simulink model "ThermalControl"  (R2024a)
settings: Solver=FixedStepDiscrete  StartTime=0.0  StopTime=10000  FixedStep=0.1  RelTol=1e-3
undefined symbols (not defined in the file): CtrlThrBattTrgTemp, CtrlThrEMTrgTemp
libraries: simulink x1

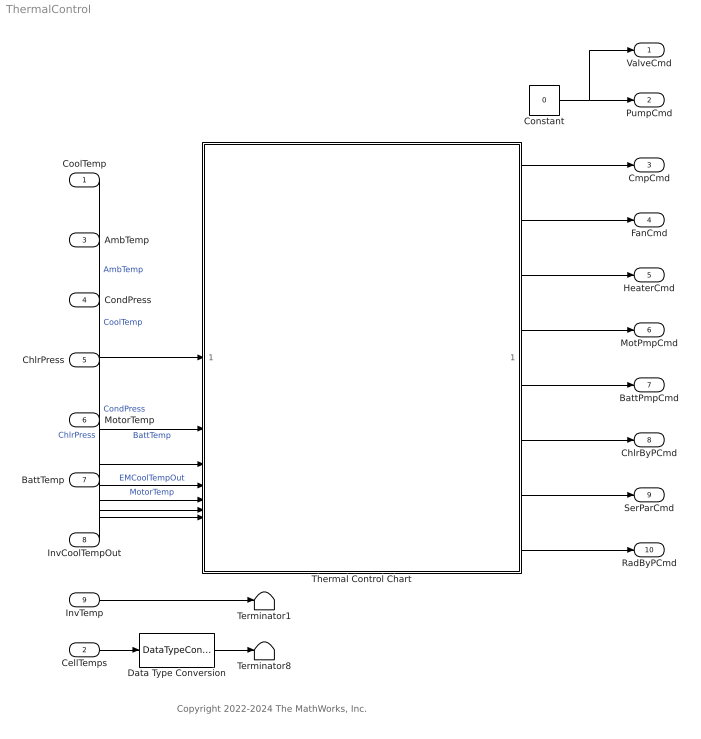
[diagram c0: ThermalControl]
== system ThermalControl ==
  note: Copyright 2022-2024 The MathWorks, Inc.
  CoolTemp : Inport  Unit=K
  CellTemps : Inport  Port=2  PortDimensions=PlntBattNumCellSer
  AmbTemp : Inport  Port=3  Unit=K
  CondPress : Inport  Port=4  Unit=MPa
  ChlrPress : Inport  Port=5  Unit=MPa
  MotorTemp : Inport  Port=6  Unit=K
  BattTemp : Inport  Port=7  Unit=K
  InvCoolTempOut : Inport  Port=8  Unit=K
  InvTemp : Inport  Port=9  Unit=K
  Constant : Constant  Value=0  SampleTime=0.1
  Data Type Conversion : DataTypeConversion  OutDataTypeStr=single
  Terminator1 : Terminator
  Terminator8 : Terminator
  Thermal Control Chart : Stateflow chart  TreatAsAtomicUnit=on
  ValveCmd : Outport
  PumpCmd : Outport  Port=2
  CmpCmd : Outport  Port=3
  FanCmd : Outport  Port=4
  HeaterCmd : Outport  Port=5
  MotPmpCmd : Outport  Port=6
  BattPmpCmd : Outport  Port=7
  ChlrByPCmd : Outport  Port=8
  SerParCmd : Outport  Port=9
  RadByPCmd : Outport  Port=10
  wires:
  AmbTemp/1 -> Thermal Control Chart/1(AmbTemp)  "AmbTemp"
  CondPress/1 -> Thermal Control Chart/7(CondPress)  "CondPress"
  BattTemp/1 -> Thermal Control Chart/2(BattTemp)  "BattTemp"
  InvCoolTempOut/1 -> Thermal Control Chart/4(EMCoolTempOut)  "EMCoolTempOut"
  CoolTemp/1 -> Thermal Control Chart/3(CoolTemp)  "CoolTemp"
  MotorTemp/1 -> Thermal Control Chart/5(MotorTemp)  "MotorTemp"
  Thermal Control Chart/1(BattPmpCmd) -> BattPmpCmd/1
  Thermal Control Chart/2(ChlrByPCmd) -> ChlrByPCmd/1
  Thermal Control Chart/5(MotPmpCmd) -> MotPmpCmd/1
  Thermal Control Chart/4(SerParCmd) -> SerParCmd/1
  Thermal Control Chart/3(RadByPCmd) -> RadByPCmd/1
  Thermal Control Chart/6(HeaterCmd) -> HeaterCmd/1
  Thermal Control Chart/7(CmpCmd) -> CmpCmd/1
  ChlrPress/1 -> Thermal Control Chart/6(ChlrPress)  "ChlrPress"
  Thermal Control Chart/8(FanCmd) -> FanCmd/1
  Constant/1 -> ValveCmd/1, PumpCmd/1
  Data Type Conversion/1 -> Terminator8/1
  CellTemps/1 -> Data Type Conversion/1
  InvTemp/1 -> Terminator1/1

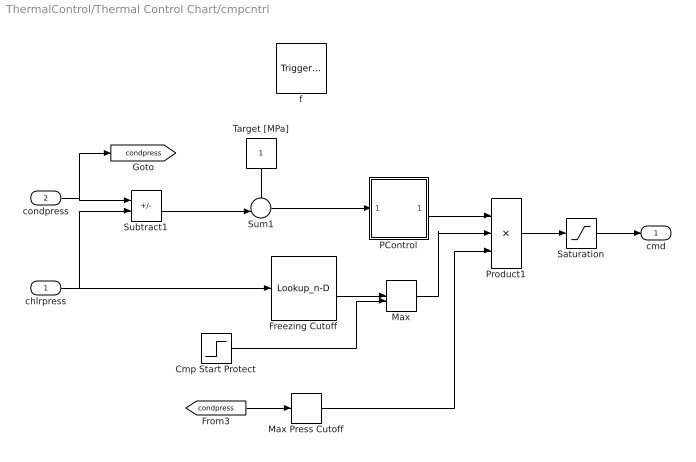
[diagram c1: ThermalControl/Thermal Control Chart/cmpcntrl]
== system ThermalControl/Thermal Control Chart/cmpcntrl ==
  chlrpress : Inport  OutDataTypeStr=double  PortDimensions=1
  condpress : Inport  Port=2  OutDataTypeStr=double  PortDimensions=1
  f : TriggerPort  TriggerType=function-call  VariantControl=(inherit)  SampleTime=-1
  Cmp Start Protect : Step  Time=15  Before=1  After=0
  Freezing Cutoff : Lookup_n-D  NumberOfTableDimensions=1  BreakpointsForDimension1=[0.3 0.31]  IndexSearchMethod=Linear search  BeginIndexSearchUsingPreviousIndexResult=on  Table=[0.1 1]  ExtrapMethod=Clip  InternalRulePriority=Speed  RndMeth=Simplest
  Max : MinMax  Function=max  Inputs=2
  Max Press Cutoff : Relay  OnSwitchValue=3  OffSwitchValue=2.9  OnOutputValue=0.1  OffOutputValue=1
  PControl : Subsystem
  Product1 : Product  Inputs=3
  Saturation : Saturate  UpperLimit=1  LowerLimit=0.1
  Subtract1 : Sum  Inputs=+-
  Sum1 : Sum  Inputs=+-|
  Target [MPa] : Constant
  cmd : Outport
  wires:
  Target [MPa]/1 -> Sum1/1
  Cmp Start Protect/1 -> Max/2
  Max/1 -> Product1/2
  Saturation/1 -> cmd/1
  PControl/1(cmd) -> Product1/1
  [condpress] -> Max Press Cutoff/1
  Max Press Cutoff/1 -> Product1/3
  Freezing Cutoff/1 -> Max/1
  Sum1/1 -> PControl/1(input)
  Product1/1 -> Saturation/1
  Subtract1/1 -> Sum1/2
  condpress/1 -> [condpress], Subtract1/1
  chlrpress/1 -> Subtract1/2, Freezing Cutoff/1

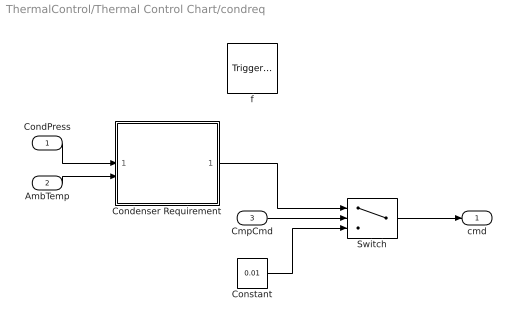
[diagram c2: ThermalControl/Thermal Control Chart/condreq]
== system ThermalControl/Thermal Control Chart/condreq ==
  CondPress : Inport  OutDataTypeStr=double  PortDimensions=1
  AmbTemp : Inport  Port=2  OutDataTypeStr=double  PortDimensions=1
  CmpCmd : Inport  Port=3  OutDataTypeStr=double  PortDimensions=1
  f : TriggerPort  TriggerType=function-call  VariantControl=(inherit)  SampleTime=-1
  Condenser Requirement : Subsystem
  Constant : Constant  Value=0.01  SampleTime=-1
  Switch : Switch  Criteria=u2 > Threshold
  cmd : Outport
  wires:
  Switch/1 -> cmd/1
  Constant/1 -> Switch/3
  CmpCmd/1 -> Switch/2
  Condenser Requirement/1(cmd_fan) -> Switch/1
  CondPress/1 -> Condenser Requirement/1(p_cond)
  AmbTemp/1 -> Condenser Requirement/2(T_env)

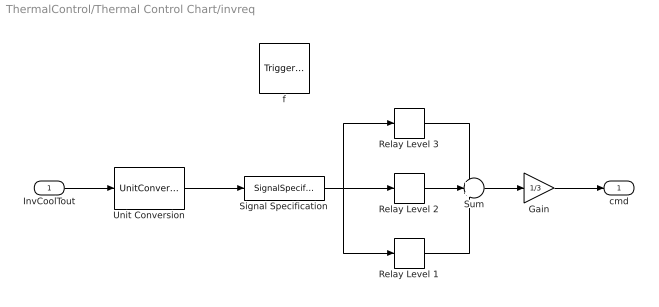
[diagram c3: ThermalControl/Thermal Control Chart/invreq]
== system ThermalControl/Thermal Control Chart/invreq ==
  InvCoolTout : Inport  OutDataTypeStr=double  Unit=K  PortDimensions=1
  f : TriggerPort  TriggerType=function-call  VariantControl=(inherit)  SampleTime=-1
  Gain : Gain  Gain=1/3
  Relay Level 1 : Relay  OnSwitchValue=75  OffSwitchValue=65
  Relay Level 2 : Relay  OnSwitchValue=85  OffSwitchValue=76
  Relay Level 3 : Relay  OnSwitchValue=95  OffSwitchValue=86
  Signal Specification : SignalSpecification  Unit=°C
  Sum : Sum  Inputs=+++
  Unit Conversion : UnitConversion
  cmd : Outport
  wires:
  Relay Level 2/1 -> Sum/2
  Sum/1 -> Gain/1
  Signal Specification/1 -> Relay Level 2/1, Relay Level 3/1, Relay Level 1/1
  Relay Level 1/1 -> Sum/3
  Relay Level 3/1 -> Sum/1
  Unit Conversion/1 -> Signal Specification/1
  Gain/1 -> cmd/1
  InvCoolTout/1 -> Unit Conversion/1

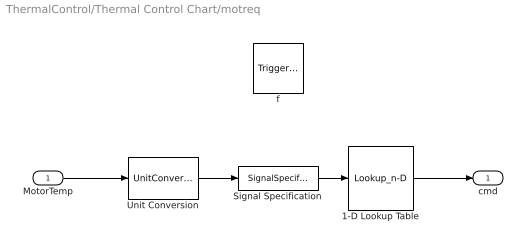
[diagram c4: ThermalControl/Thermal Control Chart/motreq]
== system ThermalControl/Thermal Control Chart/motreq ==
  MotorTemp : Inport  OutDataTypeStr=double  Unit=K  PortDimensions=1
  f : TriggerPort  TriggerType=function-call  VariantControl=(inherit)  SampleTime=-1
  1-D Lookup Table : Lookup_n-D  NumberOfTableDimensions=1  BreakpointsForDimension1=[-50 45 48 52 58 60 75 130]  IndexSearchMethod=Linear search  BeginIndexSearchUsingPreviousIndexResult=on  Table=[0 0 0.1 0.3 0.5 0.7 1 1]  InternalRulePriority=Speed  RndMeth=Simplest
  Signal Specification : SignalSpecification  Unit=°C
  Unit Conversion : UnitConversion
  cmd : Outport
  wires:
  Unit Conversion/1 -> Signal Specification/1
  Signal Specification/1 -> 1-D Lookup Table/1
  1-D Lookup Table/1 -> cmd/1
  MotorTemp/1 -> Unit Conversion/1

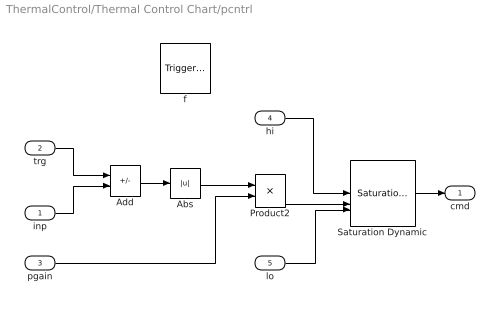
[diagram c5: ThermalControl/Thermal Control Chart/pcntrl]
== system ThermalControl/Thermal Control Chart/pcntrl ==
  inp : Inport  OutDataTypeStr=double  PortDimensions=1
  trg : Inport  Port=2  OutDataTypeStr=double  PortDimensions=1
  pgain : Inport  Port=3  OutDataTypeStr=double  PortDimensions=1
  hi : Inport  Port=4  OutDataTypeStr=double  PortDimensions=1
  lo : Inport  Port=5  OutDataTypeStr=double  PortDimensions=1
  f : TriggerPort  TriggerType=function-call  VariantControl=(inherit)  SampleTime=-1
  Abs : Abs
  Add : Sum  Inputs=+-
  Product2 : Product
  Saturation Dynamic : simulink/Discontinuities/Saturation Dynamic  OutMin=[]  OutMax=[]  OutDataTypeStr=Inherit: Same as second input  OutDataType=fixdt(1, 16)  OutScaling=2^-10  DoSatur=off
  cmd : Outport
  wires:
  trg/1 -> Add/1
  inp/1 -> Add/2
  Add/1 -> Abs/1
  Saturation Dynamic/1 -> cmd/1
  pgain/1 -> Product2/2
  Product2/1 -> Saturation Dynamic/2
  Abs/1 -> Product2/1
  hi/1 -> Saturation Dynamic/1
  lo/1 -> Saturation Dynamic/3

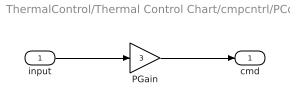
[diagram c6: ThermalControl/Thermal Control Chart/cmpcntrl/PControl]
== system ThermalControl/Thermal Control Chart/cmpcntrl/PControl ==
  input : Inport
  PGain : Gain  Gain=3
  cmd : Outport
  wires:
  input/1 -> PGain/1
  PGain/1 -> cmd/1

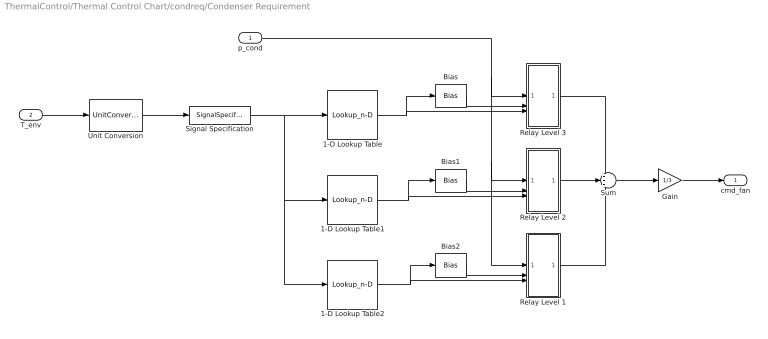
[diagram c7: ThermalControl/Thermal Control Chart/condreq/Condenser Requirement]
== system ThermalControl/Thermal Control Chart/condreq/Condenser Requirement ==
  p_cond : Inport
  T_env : Inport  Port=2  Unit=K
  1-D Lookup Table : Lookup_n-D  NumberOfTableDimensions=1  BreakpointsForDimension1=[0 20 30 40 50]  IndexSearchMethod=Linear search  BeginIndexSearchUsingPreviousIndexResult=on  Table=[2.0 2.0 1.8 1.5 1.3]  InternalRulePriority=Speed  RndMeth=Simplest
  1-D Lookup Table1 : Lookup_n-D  NumberOfTableDimensions=1  BreakpointsForDimension1=[0 20 30 40 50]  IndexSearchMethod=Linear search  BeginIndexSearchUsingPreviousIndexResult=on  Table=[1.4 1.4 1.3 1.2 1.1]  InternalRulePriority=Speed  RndMeth=Simplest
  1-D Lookup Table2 : Lookup_n-D  NumberOfTableDimensions=1  BreakpointsForDimension1=[0 20 30 40 50]  IndexSearchMethod=Linear search  BeginIndexSearchUsingPreviousIndexResult=on  Table=[0.8 0.8 0.8 0.8 0.8]  InternalRulePriority=Speed  RndMeth=Simplest
  Bias : Bias  Bias=0.4
  Bias1 : Bias  Bias=0.4
  Bias2 : Bias  Bias=0.3
  Gain : Gain  Gain=1/3
  Relay Level 1 : Subsystem
  Relay Level 2 : Subsystem
  Relay Level 3 : Subsystem
  Signal Specification : SignalSpecification  Unit=°C
  Sum : Sum  Inputs=+++
  Unit Conversion : UnitConversion
  cmd_fan : Outport
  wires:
  Unit Conversion/1 -> Signal Specification/1
  Signal Specification/1 -> 1-D Lookup Table2/1, 1-D Lookup Table1/1, 1-D Lookup Table/1
  Gain/1 -> cmd_fan/1
  T_env/1 -> Unit Conversion/1
  Bias2/1 -> Relay Level 1/2(high)
  1-D Lookup Table2/1 -> Bias2/1, Relay Level 1/3(low)
  Bias1/1 -> Relay Level 2/2(high)
  1-D Lookup Table1/1 -> Bias1/1, Relay Level 2/3(low)
  Bias/1 -> Relay Level 3/2(high)
  1-D Lookup Table/1 -> Bias/1, Relay Level 3/3(low)
  Relay Level 1/1(out) -> Sum/3
  Relay Level 2/1(out) -> Sum/2
  Relay Level 3/1(out) -> Sum/1
  p_cond/1 -> Relay Level 1/1(in), Relay Level 2/1(in), Relay Level 3/1(in)
  Sum/1 -> Gain/1

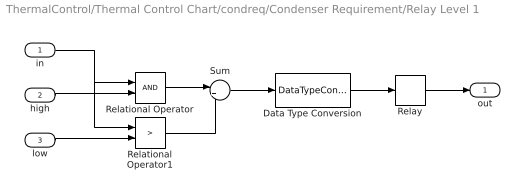
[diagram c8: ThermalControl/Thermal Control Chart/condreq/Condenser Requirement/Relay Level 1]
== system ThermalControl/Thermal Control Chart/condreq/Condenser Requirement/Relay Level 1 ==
  in : Inport
  high : Inport  Port=2
  low : Inport  Port=3
  Data Type Conversion : DataTypeConversion
  Relational Operator : RelationalOperator  OutDataTypeStr=boolean  RndMeth=Simplest
  Relational Operator1 : RelationalOperator  Operator=>  OutDataTypeStr=boolean  RndMeth=Simplest
  Relay : Relay  OnSwitchValue=1.5  OffSwitchValue=0.5
  Sum : Sum  Inputs=|++
  out : Outport
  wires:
  in/1 -> Relational Operator1/1, Relational Operator/1
  high/1 -> Relational Operator/2
  low/1 -> Relational Operator1/2
  Relay/1 -> out/1
  Relational Operator/1 -> Sum/1
  Relational Operator1/1 -> Sum/2
  Data Type Conversion/1 -> Relay/1
  Sum/1 -> Data Type Conversion/1

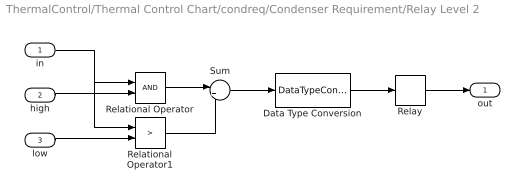
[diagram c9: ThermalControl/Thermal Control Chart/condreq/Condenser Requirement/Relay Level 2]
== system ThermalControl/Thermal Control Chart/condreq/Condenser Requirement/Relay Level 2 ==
  in : Inport
  high : Inport  Port=2
  low : Inport  Port=3
  Data Type Conversion : DataTypeConversion
  Relational Operator : RelationalOperator  OutDataTypeStr=boolean  RndMeth=Simplest
  Relational Operator1 : RelationalOperator  Operator=>  OutDataTypeStr=boolean  RndMeth=Simplest
  Relay : Relay  OnSwitchValue=1.5  OffSwitchValue=0.5
  Sum : Sum  Inputs=|++
  out : Outport
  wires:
  in/1 -> Relational Operator1/1, Relational Operator/1
  high/1 -> Relational Operator/2
  low/1 -> Relational Operator1/2
  Relay/1 -> out/1
  Relational Operator/1 -> Sum/1
  Relational Operator1/1 -> Sum/2
  Data Type Conversion/1 -> Relay/1
  Sum/1 -> Data Type Conversion/1

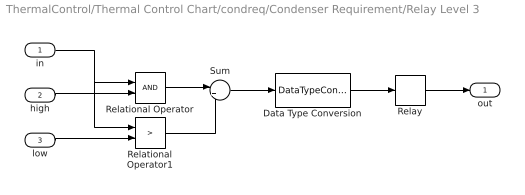
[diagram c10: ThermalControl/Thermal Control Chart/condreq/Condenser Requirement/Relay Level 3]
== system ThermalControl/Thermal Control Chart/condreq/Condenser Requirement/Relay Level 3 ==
  in : Inport
  high : Inport  Port=2
  low : Inport  Port=3
  Data Type Conversion : DataTypeConversion
  Relational Operator : RelationalOperator  OutDataTypeStr=boolean  RndMeth=Simplest
  Relational Operator1 : RelationalOperator  Operator=>  OutDataTypeStr=boolean  RndMeth=Simplest
  Relay : Relay  OnSwitchValue=1.5  OffSwitchValue=0.5
  Sum : Sum  Inputs=|++
  out : Outport
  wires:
  in/1 -> Relational Operator1/1, Relational Operator/1
  high/1 -> Relational Operator/2
  low/1 -> Relational Operator1/2
  Relay/1 -> out/1
  Relational Operator/1 -> Sum/1
  Relational Operator1/1 -> Sum/2
  Data Type Conversion/1 -> Relay/1
  Sum/1 -> Data Type Conversion/1

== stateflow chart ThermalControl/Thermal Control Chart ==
  state Pumps [parallel]
    state PumpsON
      during:
      BattPmpCmd = ...
      pcntrl(BattTemp,CtrlThrBattTrgTemp,1,1,0.1);
    state PumpsOFF
      entry:
      BattPmpCmd = 0.01;
    (default) -> PumpsOFF
    PumpsOFF -> PumpsON : [BattTemp - CtrlThrBattTrgTemp > 0 || MotorTemp - CtrlThrEMTrgTemp > 3 || ...  CtrlThrBattTrgTemp - AmbTemp > 20]
    PumpsON -> PumpsOFF : [CtrlThrBattTrgTemp - BattTemp > 5 && CtrlThrEMTrgTemp - MotorTemp > 5]
  state Heater [parallel]
    state HeatON
      entry:
      HeaterCmd = 1;
    state HeatOFF
      entry:
      HeaterCmd = 0;
    (default) -> HeatOFF
    HeatOFF -> HeatON : [BattPmpCmd > 0 && CtrlThrBattTrgTemp - CoolTemp > 20 && ... CtrlThrBattTrgTemp - AmbTemp > 20 ]
    HeatON -> HeatOFF : [CtrlThrBattTrgTemp - CoolTemp < 10]
  state cmd = pcntrl(inp,trg,pgain,hi,lo) [function]
  state cmd = cmpcntrl(chlrpress, ... [function]
    condpress)
  state ChillerBypass [parallel]
    state ChillerON
      entry:
      ChlrByPCmd = 0;
      during:
      CmpCmd = ...
      cmpcntrl(ChlrPress,CondPress);
    state ChillerOFF
      entry:
      ChlrByPCmd = 1;
      CmpCmd = 0;
    (default) -> ChillerOFF
    ChillerOFF -> ChillerON : [HeaterCmd == 0 && BattPmpCmd > 0.01 && ...  BattTemp - CtrlThrBattTrgTemp > 0 && ... BattTemp - CoolTemp < 5]
    ChillerON -> ChillerOFF : [CtrlThrBattTrgTemp - BattTemp > 5 ]
  state cmd = condreq(CondPress, ... [function]
    AmbTemp,CmpCmd)
  state cmd = invreq(InvCoolTout) [function]
  state RadiatorBypass [parallel]
    state RadiatorON
      entry:
      RadByPCmd = 0;
      during:
      fcmd1 = condreq(CondPress,AmbTemp,CmpCmd);
      fcmd2 = invreq(EMCoolTempOut);
      fcmd3 = motreq(MotorTemp);
      FanCmd = max([fcmd1,fcmd2,fcmd3]);
    state RadiatorOFF
      entry:
      RadByPCmd = 1;
      during:
      FanCmd = condreq(CondPress,AmbTemp,CmpCmd);
    (default) -> RadiatorOFF
    RadiatorOFF -> RadiatorON : [HeaterCmd == 0 && BattPmpCmd > 0 && ... EMCoolTempOut - CtrlThrEMTrgTemp > 0 && ... EMCoolTempOut - AmbTemp > 0]
    RadiatorON -> RadiatorOFF : [AmbTemp - EMCoolTempOut > 0]
  state cmd = motreq(MotorTemp) [function]
  state SeriesParallel [parallel]
    state Parallel
      entry:
      SerParCmd = 0;
      during:
      MotPmpCmd = ...
      pcntrl(MotorTemp,CtrlThrEMTrgTemp,1,1,0.1);
    state Series
      entry:
      SerParCmd = 1;
      during:
      MotPmpCmd = BattPmpCmd;
    (default) -> Series
    Series -> Parallel : [BattPmpCmd > 0.01 && (ChlrByPCmd < 0.5 || ... max(AmbTemp,EMCoolTempOut) - CtrlThrBattTrgTemp > 10 ... || MotorTemp - BattTemp > 50)]
    Parallel -> Series : [max(AmbTemp,EMCoolTempOut) - CtrlThrBattTrgTemp < 5]
  data: inp function_input double; trg function_input double; pgain function_input double; hi function_input double; lo function_input double; cmd function_output; chlrpress function_input double; condpress function_input double; cmd function_output; CondPress function_input double; AmbTemp function_input double; CmpCmd function_input double; cmd function_output; InvCoolTout function_input double; cmd function_output; MotorTemp function_input double; cmd function_output; AmbTemp input double; BattTemp input; CoolTemp input; EMCoolTempOut input; MotorTemp input double; BattPmpCmd output; ChlrByPCmd output; RadByPCmd output; SerParCmd output; MotPmpCmd output; HeaterCmd output; CtrlThrBattTrgTemp parameter; CtrlThrEMTrgTemp parameter; CmpCmd output double; ChlrPress input; CondPress input double; FanCmd output double; fcmd1 local; fcmd2 local; fcmd3 local
